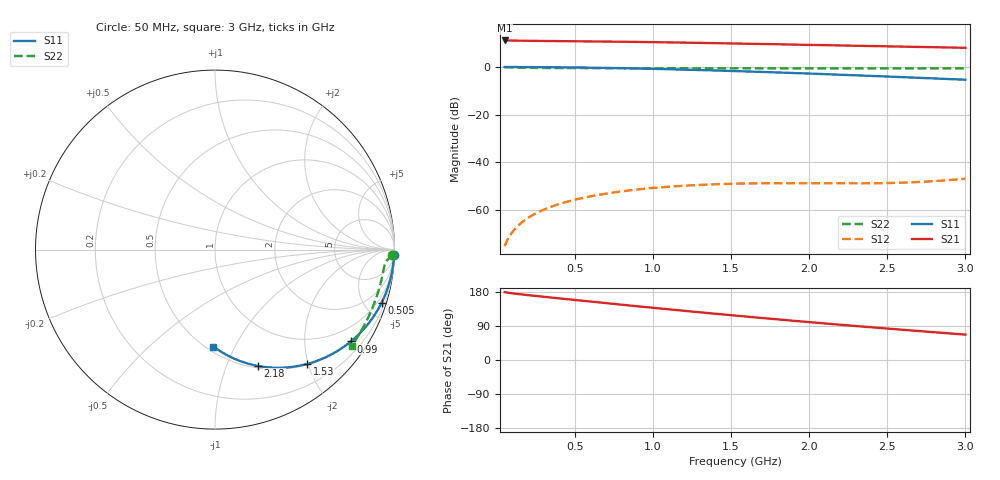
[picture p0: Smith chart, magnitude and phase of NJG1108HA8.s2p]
!	NJG1108HA8 Spar
#	mhz	S	ma	R	50
!	2	Port	Network	Data	from	SP1.SP	block
!	freq	magS11	angS11	magS21	angS21	magS12	angS12	magS22	angS22
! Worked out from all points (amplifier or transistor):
!   591 points, 50 MHz to 3 GHz, reference 50 ohm
!   highest |S21| = 11.1 dB at 50 MHz (marker M1)
!   |S21| within 3 dB of that: start of sweep to 2.932 GHz
!   unconditionally stable (mu >= 1): 850.6 MHz to end of sweep
!   at 540 MHz: K = 0.62, MSG = 32.9 dB, |S12| = -55.0 dB
!   at 1.525 GHz: K = 2.01, MAG = 23.6 dB, |S12| = -48.9 dB
!   at 3 GHz: K = 3.80, MAG = 18.7 dB, |S12| = -46.8 dB
!   lowest NFmin = 0.26 dB at 50 MHz
!   S11 on the Smith chart (normalised r, x): 50 MHz: 5, -64; 505 MHz: 0.55, -6.38; 990 MHz: 0.51, -3.19; 1.53 GHz: 0.51, -1.99; 2.18 GHz: 0.52, -1.30; 3 GHz: 0.54, -0.83
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50  0.9975 -1.8  3.588 179.1  0.0001762 89.1  0.9881 -1.7
85  0.997 -3.0  3.57 176.7  0.000298 88.0  0.9785 -2.4
115  0.9964 -4.1  3.555 175.1  0.0004014 87.2  0.971 -2.9
155  0.9954 -5.5  3.538 173.2  0.000538 86.4  0.9635 -3.3
205  0.9937 -7.2  3.523 171.0  0.0007072 85.5  0.9573 -3.7
265  0.9911 -9.3  3.509 168.4  0.0009078 84.4  0.9529 -4.3
335  0.9872 -11.8  3.494 165.4  0.001138 83.1  0.9499 -4.9
505  0.9743 -17.7  3.457 158.2  0.001671 80.0  0.9462 -6.6
545  0.9705 -19.1  3.448 156.5  0.001791 79.4  0.9456 -7.0
775  0.9444 -26.9  3.384 146.9  0.002417 75.6  0.9431 -9.5
990  0.9137 -34.0  3.312 138.1  0.002897 72.7  0.9412 -11.9
1035  0.9067 -35.5  3.296 136.3  0.002983 72.1  0.9408 -12.5
1155  0.887 -39.4  3.251 131.5  0.003187 70.9  0.9397 -13.8
1280  0.8652 -43.3  3.201 126.6  0.00336 69.8  0.9387 -15.2
1525  0.8199 -50.9  3.099 117.3  0.003585 68.9  0.9367 -18.0
1530  0.8189 -51.0  3.097 117.1  0.003588 68.9  0.9367 -18.1
1770  0.7724 -58.1  2.995 108.2  0.003675 69.7  0.935 -20.8
2020  0.7231 -65.2  2.889 99.3  0.003671 73.0  0.9335 -23.7
2180  0.6917 -69.6  2.822 93.7  0.00365 76.7  0.9328 -25.5
2510  0.6283 -78.4  2.691 82.6  0.003703 88.4  0.9318 -29.4
2765  0.5813 -85.0  2.597 74.3  0.003992 100.0  0.9316 -32.4
3000  0.5401 -90.9  2.517 67.0  0.004558 110.4  0.9317 -35.3
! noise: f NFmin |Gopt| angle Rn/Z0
50  0.2602  0.9589  4.081  1.429
375  0.2868  0.8907  9.092  0.5703
705  0.3435  0.8661  15.8  0.5467
1030  0.417  0.8355  22.76  0.5241
1360  0.5008  0.7997  30.02  0.4956
1685  0.5878  0.7608  37.36  0.4622
2015  0.6784  0.7181  45.04  0.4237
2340  0.7684  0.6729  52.86  0.3827
2670  0.8599  0.6238  61.12  0.3394
3000  0.9508  0.5715  69.79  0.2961
